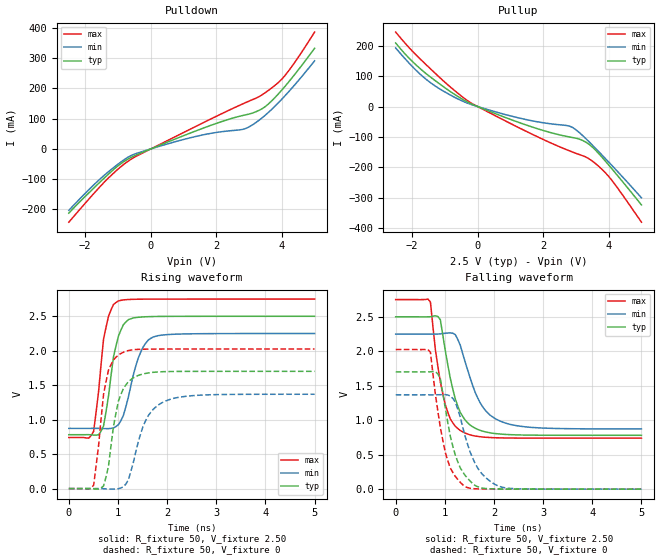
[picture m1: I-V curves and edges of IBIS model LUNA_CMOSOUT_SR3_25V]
[IBIS Ver]   3.2
[Comment Char]   |_char
[File name]   sg2016cba_25v_b.ibs
[File Rev]   1.1
[Date]   2025/6/20 10:41:50
[Source]
[Notes]
[Disclaimer]
This information is for modeling purposes only, and is not guaranteed.
Property of SEIKO EPSON Corp.,
unauthorized reproduction and/or distribution is strictly prohibited.
[Copyright]
Copyright 2021, SEIKO EPSON Corp.
[Component]   2G005_2016
Si_location Pin
Timing_location Pin
[Manufacturer]   SEIKO EPSON Corp.
| 2016 PKG
[Package]
R_pkg   25m   NA   NA
L_pkg   0.25n   NA   NA
C_pkg   0.183p   NA   NA
[Pin] signal_name   model_name
1   OE   NC
2   GND   GND
3   OUT   LUNA_CMOSOUT_SR3_25V
4   VCC   POWER
| Models and submodels in the file (1): LUNA_CMOSOUT_SR3_25V (Output)
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[Model]   LUNA_CMOSOUT_SR3_25V
Model_type Output
Polarity Non-Inverting
Vmeas=1.25
C_comp   2.5p   2.0p   3.0p
[Temperature Range] 25   140   -40
[Voltage Range]   2.50   2.25   2.75
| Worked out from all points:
|   slope of the pulldown table from 0 to 0.375 V, typ, clamps not added: 22.6 ohm
|   slope of the pullup table from 0 to 0.375 V, typ, clamps not added: 23.1 ohm
|   falling waveform, R_fixture 50, V_fixture 2.50: 20-80 % time 331ps typ, 457ps min, 289ps max; typ from 2.5 V to 0.782 V
|   falling waveform, R_fixture 50, V_fixture 0: 20-80 % time 330ps typ, 407ps min, 298ps max; typ from 1.7 V to 0 V
|   rising waveform, R_fixture 50, V_fixture 2.50: 20-80 % time 231ps typ, 315ps min, 199ps max; typ from 0.782 V to 2.5 V
|   rising waveform, R_fixture 50, V_fixture 0: 20-80 % time 247ps typ, 382ps min, 209ps max; typ from 0 V to 1.7 V
[Pullup]
-2.5V     208.9mA    192.4mA    244.7mA
-2.1V     159.8mA    143.6mA    194.6mA
-1.6V     110.5mA    91.96mA    140.5mA
-1.1V     69.63mA    54.27mA    89.78mA
-500mV    26.23mA    19.76mA    34.8mA
-100mV    4.416mA    3.368mA    5.668mA
1.4V      -57.68mA   -40.98mA   -77.15mA
2.9V      -102mA     -68.96mA   -149.8mA
3.4V      -124mA     -115.8mA   -171.7mA
3.9V      -179.5mA   -171.1mA   -217.8mA
4.2V      -217.9mA   -205.4mA   -257.3mA
5V        -323.4mA   -300.1mA   -380.1mA
[Pulldown]
-2.5V     -212.5mA   -203.1mA   -242.3mA
-1.4V     -94.37mA   -85.35mA   -107.9mA
-1V       -56.04mA   -50.51mA   -66.89mA
-600mV    -27.76mA   -21.78mA   -33.9mA
600mV     26.47mA    19.32mA    32.57mA
1.7V      72.74mA    48.79mA    91.95mA
2.8V      110.4mA    64.5mA     148.6mA
3.1V      118.4mA    79.21mA    162.8mA
3.5V      140.4mA    112mA      186.4mA
4V        194.7mA    164.5mA    230.8mA
4.4V      247.2mA    212.7mA    287.1mA
5V        333mA      291.5mA    386.4mA
[Falling Waveform]
R_fixture=50
V_fixture=2.50
V_fixture_min=2.25
V_fixture_max=2.75
0s        2.5V       2.25V      2.75V
707.1ps   2.501V     2.25V      2.713V
808.1ps   2.515V     2.249V     2.02V
909.1ps   2.456V     2.252V     1.552V
1.01ns    2.006V     2.261V     1.222V
1.162ns   1.453V     2.262V     962.7mV
1.313ns   1.114V     2.089V     851mV
1.717ns   852.8mV    1.254V     760.9mV
2.121ns   800.2mV    988.6mV    744.3mV
5ns       781.6mV    873.5mV    740.4mV
[Falling Waveform]
R_fixture=50
V_fixture=0
V_fixture_min=0
V_fixture_max=0
0s        1.701V     1.369V     2.025V
707.1ps   1.702V     1.368V     1.984V
808.1ps   1.705V     1.368V     1.372V
909.1ps   1.604V     1.371V     892.4mV
1.01ns    1.172V     1.372V     530.1mV
1.212ns   494.7mV    1.265V     185.7mV
1.414ns   198.3mV    762.5mV    35.11mV
1.717ns   22.51mV    254mV      3.221mV
2.121ns   2.668mV    37.51mV    1.12mV
5ns       304.7uV    564.5uV    186.4uV
[Rising Waveform]
R_fixture=50
V_fixture=2.50
V_fixture_min=2.25
V_fixture_max=2.75
0s        781.6mV    873.3mV    740.4mV
505.1ps   776.8mV    873.6mV    831.3mV
707.1ps   909.1mV    871.2mV    2.171V
808.1ps   1.343V     869.5mV    2.502V
909.1ps   1.912V     880.3mV    2.671V
1.01ns    2.213V     927.9mV    2.724V
1.111ns   2.378V     1.063V     2.738V
1.414ns   2.486V     1.897V     2.748V
1.717ns   2.496V     2.2V       2.749V
5ns       2.5V       2.25V      2.75V
[Rising Waveform]
R_fixture=50
V_fixture=0
V_fixture_min=0
V_fixture_max=0
0s        0V         0V         0V
505.1ps   -3.751mV   252.1uV    49.13mV
707.1ps   39.05mV    -1.781mV   1.369V
757.6ps   169.9mV    -3.994mV   1.554V
909.1ps   904.7mV    -8.506mV   1.868V
1.061ns   1.367V     9.462mV    1.96V
1.212ns   1.552V     126.6mV    2.003V
1.566ns   1.671V     989mV      2.023V
1.919ns   1.696V     1.254V     2.025V
5ns       1.701V     1.369V     2.025V
[Ramp]
R_load=50
dV/dt_r   1.021E+0/2.471E-10   8.212E-1/3.816E-10   1.215E+0/2.069E-10
dV/dt_f   1.031E+0/3.280E-10   8.259E-1/4.570E-10   1.206E+0/2.887E-10
|[End   LUNA_CMOSOUT_SR3_25V
